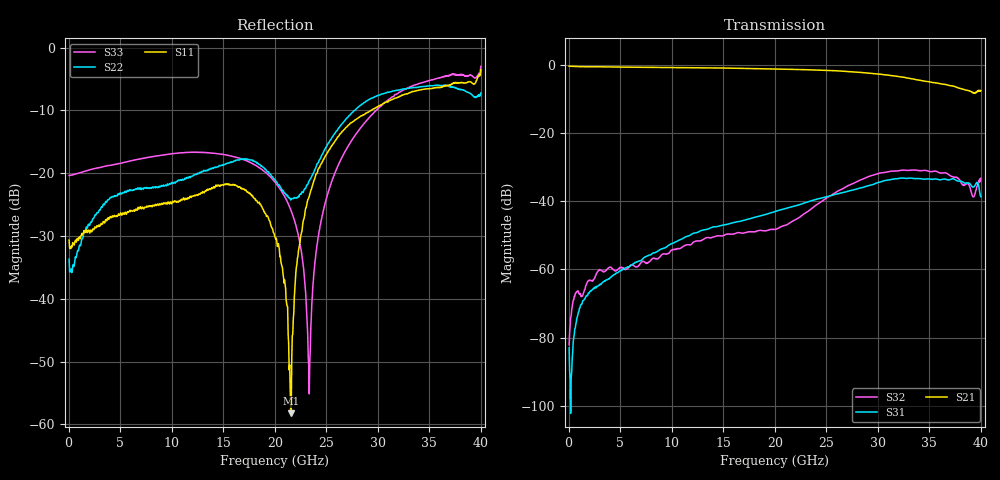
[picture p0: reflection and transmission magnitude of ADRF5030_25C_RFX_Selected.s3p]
! Device  : ADRF5030
! Description: Silicon SPDT Switch Non-Reflective
! Frequency:  100 MHz -  20 GHz
! Ports:
!  RFC = Port 1
!  RF1 = Port 2
!  RF2 = Port 3
! VSS  =  -3.30 Volts
! VDD  =  +3.30 Volts
! EN  =  0.00 Volts
! LS  =  0.00 Volts
! V1  =  +3.30 Volts
! Data:  Data was collected using an calibrated 4 port network analyzer.
! Notes: Analog Devices supplies this data as a sample of measured data
!  for this product.  Your particular data for this product may vary.
!  Data was taken at +25 degrees C.
!  Analog Devices reserves the right to change this data at anytime.
# HZ S DB R 50
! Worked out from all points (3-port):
!   800 points, 50 MHz to 40 GHz, reference 50 ohm
!   strongest paths, dB at 50 MHz, 10.05 GHz, 20.05 GHz, 30.05 GHz, 40 GHz:
!     S21: -0.4, -0.8, -1.3, -2.7, -7.6
!     S31: -83.0, -52.3, -43.0, -34.5, -38.7
!     S32: -82.1, -54.2, -48.2, -31.9, -33.2
!   lowest |S11| = -58.2 dB at 21.55 GHz (marker M1), VSWR 1.00, Z = 50 + j0.122 ohm
!   |S11| at or under -10 dB: start of sweep to 29.37 GHz
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5e7  -30.68 -3.8  -0.42 -0.2  -82.98 -34.9
     -0.42 -0.2  -33.69 -11.8  -82.07 -43.3
     -82.98 -34.9  -82.07 -43.3  -20.38 0.3
7.9e9  -25.34 139.1  -0.74 -101.5  -55.75 73.5
       -0.74 -101.5  -22.38 -143.7  -57.58 120.8
       -55.75 73.5  -57.58 120.8  -17.43 -85.1
1.395e10  -22.45 5.2  -0.92 -179.8  -47.58 48.4
          -0.92 -179.8  -19.18 -156.8  -50.57 48.4
          -47.58 48.4  -50.57 48.4  -16.82 -136.3
2.005e10  -30.22 -105.8  -1.26 98.2  -43.04 0.6
          -1.26 98.2  -21.10 165.6  -48.20 -44.3
          -43.04 0.6  -48.20 -44.3  -21.45 175.1
2.155e10  -58.24 90.4  -1.35 76.9  -41.76 -18.4
          -1.35 76.9  -24.28 -175.6  -46.19 -79.5
          -41.76 -18.4  -46.19 -79.5  -25.79 164.2
2.335e10  -23.70 37.3  -1.48 50.5  -40.06 -43.4
          -1.48 50.5  -21.23 -141.2  -42.70 -121.9
          -40.06 -43.4  -42.70 -121.9  -55.15 -114.3
2.53e10  -16.21 0.0  -1.68 21.9  -38.48 -74.7
         -1.68 21.9  -14.98 -139.9  -38.57 -159.1
         -38.48 -74.7  -38.57 -159.1  -22.38 -53.5
3.09e10  -8.68 -82.1  -3.01 -54.6  -33.87 -156.6
         -3.01 -54.6  -7.13 153.0  -31.43 118.0
         -33.87 -156.6  -31.43 118.0  -8.47 -118.2
3.645e10  -6.08 -155.2  -5.73 -125.2  -33.47 126.0
          -5.73 -125.2  -6.00 74.3  -31.69 38.6
          -33.47 126.0  -31.69 38.6  -4.58 162.4
4e10  -3.53 78.1  -7.58 132.1  -38.67 39.0
      -7.58 132.1  -7.22 -63.4  -33.25 -76.2
      -38.67 39.0  -33.25 -76.2  -2.96 23.0
